TYPE dut_OP_INPUT :
STRUCT
	I600_00			:BOOL;	//	MS8_HC_ExhPress_LOW_ALARM
	I600_01			:BOOL;	//	MS8_HC_ExhPress_HIGH_ALARM
	I600_02			:BOOL;	//	MS1_Heater_ExhPress_LOW_ALARM
	I600_03			:BOOL;	//	MS1_Heater_ExhPress_HIGH_ALARM
	I600_04			:BOOL;	//	MS3_Scavenger_ExhPress_LOW_ALARM
	I600_05			:BOOL;	//	MS3_Scavenger_ExhPress_HIGH_ALARM
	I600_06			:BOOL;	//	MS6_Frontbody_ExhPress_LOW_ALARM
	I600_07			:BOOL;	//	MS6_Frontbody_ExhPress_HIGH_ALARM
	I600_08			:BOOL;	//	MS9_LSC1_ExhPress_LOW_ALARM
	I600_09			:BOOL;	//	MS9_LSC1_ExhPress_HIGH_ALARM
	I600_10			:BOOL;	//	MS11_GasBox_ExhPress_LOW_ALARM
	I600_11			:BOOL;	//	MS11_GasBox_ExhPress_HIGH_ALARM
	I600_12			:BOOL;	//	MS12_GasBox_ExhPress_LOW_ALARM
	I600_13			:BOOL;	//	MS12_GasBox_ExhPress_HIGH_ALARM
	I600_14			:BOOL;	//	SPARE
	I600_15			:BOOL;	//	SPARE
	
	IW600			:INT;	//	MS8_RHC_ExhPress
	IW601			:INT;	//	MS1_Heater_ExhPress
	IW602			:INT;	//	MS3_Scavenger_ExhPress
	IW603			:INT;	//	MS6_Frontbody_ExhPress
	IW604			:INT;	//	MS9_LSC1_ExhPress
	IW605			:INT;	//	MS11_GasBox_ExhPress
	IW606			:INT;	//	MS12_GasBox_ExhPress
	IW607			:INT;	//	SPARE

END_STRUCT
END_TYPE
